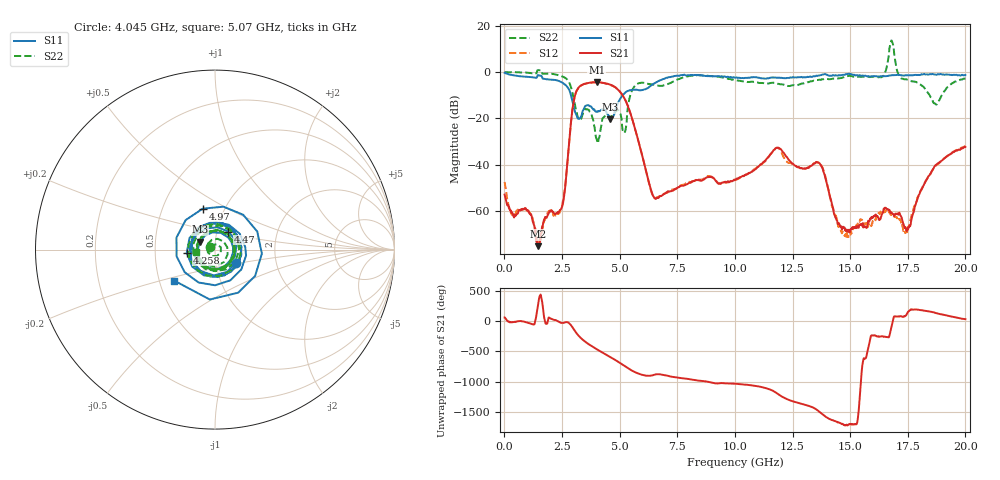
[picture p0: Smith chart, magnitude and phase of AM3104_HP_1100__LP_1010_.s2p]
!Created with skrf (http://scikit-rf.org).
# Hz S RI R 50.0
!freq ReS11 ImS11 ReS21 ImS21 ReS12 ImS12 ReS22 ImS22
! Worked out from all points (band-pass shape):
!   1601 points, 10 MHz to 20 GHz, reference 50 ohm
!   highest |S21| = -4.45 dB at 4.008 GHz (marker M1); lowest = -75.1 dB at 1.472 GHz (marker M2)
!   |S21| within 3 dB of the highest: 3.171 GHz to 4.911 GHz (1.739 GHz wide, 43 % of centre)
!   lowest |S11| = -20.4 dB at 4.595 GHz (marker M3), VSWR 1.21, Z = 42.1 + j3.7 ohm
!   |S11| at or under -10 dB: 2.889 GHz to 5.135 GHz (2.247 GHz wide, 56 % of centre)
!   |S22| runs from -30.7 to 13.6 dB; largest |S21 - S12| = 0.049
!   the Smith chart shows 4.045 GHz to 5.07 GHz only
!   S11 on the Smith chart (normalised r, x): 4.045 GHz: 1.25, -0.19; 4.258 GHz: 0.73, -0.03; 4.47 GHz: 1.14, +0.23; 4.97 GHz: 0.79, +0.38; 5.07 GHz: 0.60, -0.22
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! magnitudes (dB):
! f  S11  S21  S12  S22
! 10 MHz  -0.4  -52.9  -47.4  -0.1
! 1.472 GHz  -1.4  -75.1  -73.4  0.8
! 2.471 GHz  -4.4  -58.9  -58.5  -1.8
! 2.996 GHz  -14.5  -13.3  -13.3  -10.9
! 3.346 GHz  -18.8  -5.7  -5.8  -19.9
! 4.008 GHz  -17.0  -4.4  -4.5  -29.1
! 4.045 GHz  -17.2  -4.5  -4.5  -30.7
! 4.258 GHz  -16.0  -4.7  -4.7  -20.0
! 4.47 GHz  -18.1  -5.1  -5.1  -19.3
! 4.595 GHz  -20.4  -5.5  -5.6  -19.8
! 4.97 GHz  -12.5  -8.0  -8.1  -16.8
! 5.07 GHz  -10.9  -9.2  -9.2  -19.5
! 5.707 GHz  -7.6  -25.9  -25.9  -5.5
! 6.682 GHz  -4.0  -54.3  -53.9  -5.9
! 10.01 GHz  -2.5  -46.6  -46.7  -3.6
! 11.83 GHz  -2.5  -32.7  -32.8  -5.0
! 13.34 GHz  -2.1  -40.3  -40.2  -4.0
! 14.83 GHz  -0.9  -68.3  -71.0  -1.9
! 16.68 GHz  -1.6  -59.5  -60.0  7.2
! 17.53 GHz  -1.4  -67.5  -66.8  -3.4
! 18.69 GHz  -1.1  -40.4  -40.6  -13.6
! 20 GHz  -1.3  -32.3  -32.0  -2.8
